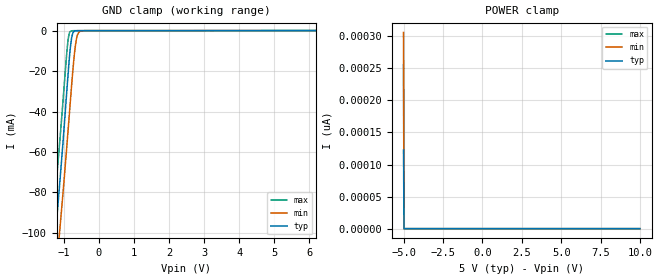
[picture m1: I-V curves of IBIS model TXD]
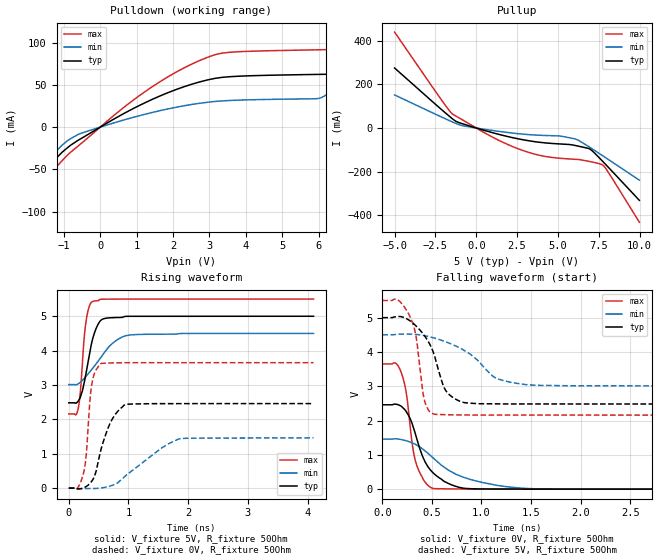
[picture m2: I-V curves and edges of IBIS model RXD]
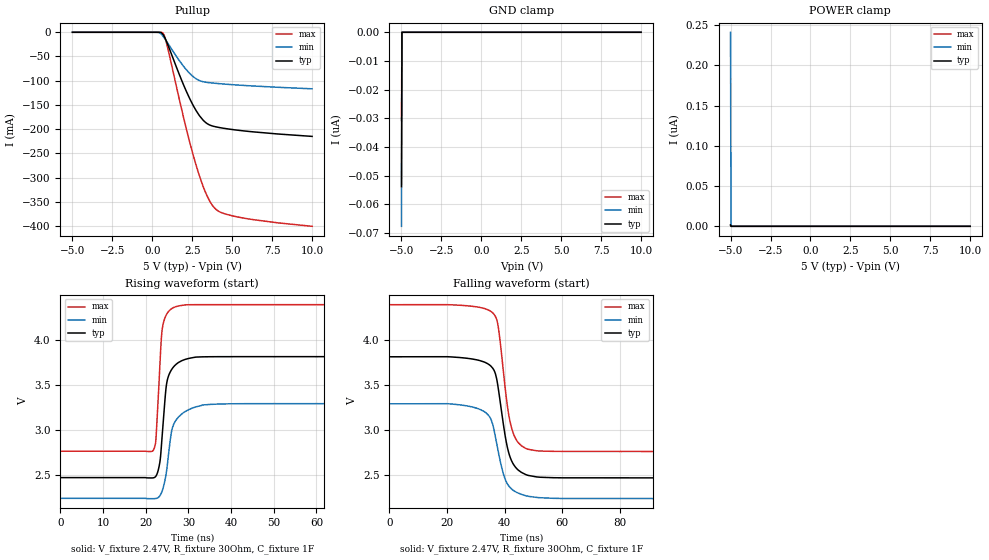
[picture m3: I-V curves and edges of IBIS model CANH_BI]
| Texas Instruments Incorporated
| CAN Transceiver Optimized for highly loaded networks
| Marketing part#   Voltage Range   Package-type   #pins/pkg drawing
| SN65HVD255D   4.5V - 5.5V   SOIC   8-pin D
[IBIS Ver]   4.0
[File name]   hvd255.ibs
[File Rev]   1.0
[Date]   05/01/2012
[Source]   Model built from TISPICED simulations at:
   Texas Instruments Incorporated.
   Analog-eLab, HPA
   12500 TI Blvd
   Dallas, TX -75243
   For Support e-mail: elab_ibis@list.ti.com
[Notes]   Revision History
   Rev 1.0: 05/01/2012
   - Initial model not matched to silicon
   - ccomp values are based on PVT settings:
   MIN: Low Voltage, High Temperature, Weak Process
   TYP: Nominal Voltage, Nominal Temperature, Nominal Process
   MAX: High Voltage, Low Temperature, Fast Process
   - User may change ccomp in the order of number values as
   per end simulator used
   - C_comp although listed in numberical order of value are obtained from varying PVT conditions.
   For PVT conditions for eachspecific value, refer to the buffer description under repective [Model].
   IBIS model user is responsible for using appropriate C_comp to simulate for Signal Integrity.
   - FAULT model not used on device HVD254
[Disclaimer] This model is designed as an aid for customers of Texas Instruments.
 TI and its licensors and suppliers make no warranties, either expressed
 or implied, with respect to this  model, including the warranties of
 merchantability or fitness for a particular purpose.
 The model is provided solely on an "as is" basis. The entire risk as to
 its quality and performance is with the customer.
[Copyright] (C)Copyright 2012 Texas Instruments Incorporated.
   All rights reserved.
|   Component HVD255D
[Component]   HVD255D
[Manufacturer]  Texas Instruments Incorporated
[Package]   |8-pin SOIC D package
|   typ   min   max
R_pkg   0.077174   0.00230   0.11690
L_pkg   2.321345nH   1.36253nH   2.80112nH
C_pkg   0.398513pF   0.31326pF   0.46592pF
[Pin] signal_name   model_name   R_pin   L_pin   C_pin
   1   TXD   TXD   0.11215   2.70023n   0.38408p
   2   GND   GND   0.03900   2.09764n   0.46592p
   3   VCC   POWER   0.02513   1.85198n   0.46577p
   4   RXD   RXD   0.11876   2.80112n   0.38992p
   5   NC   NC   0.00230   1.36253n   0.31326p
   6   CANL   CANL_BI   0.11690   2.72346n   0.40067p
   7   CANH   CANH_BI   0.09586   2.40528n   0.38694p
   8   S   S   0.10729   2.62852n   0.38154p
[Diff_pin]   inv_pin   vdiff   tdelay_typ   tdelay_min   tdelay_max
| The CANH and CANL are Diff_pins
7   6   0.9V   0 0 0
[Pin Mapping]pulldown_ref pullup_ref gnd_clamp_ref power_clamp_ref |ext_ref
1   NC   NC   GNDBUS1   PWRBUS1
2   GNDBUS1   NC
3   NC   PWRBUS1
4   GNDBUS1   PWRBUS1   GNDBUS1   PWRBUS1
5   NC   NC   NC   NC
6   GNDBUS1   NC   GNDBUS1   PWRBUS1  |CANL has no pullup
7   NC   PWRBUS1   GNDBUS1   PWRBUS1  |CANH has no pulldown
8   NC   NC   GNDBUS1   PWRBUS1
| Models and submodels in the file (6): TXD (Input), RXD (Output), CANH_BI (I/O_open_source), CANL_BI (I/O_open_drain), S (Input), FAULT (Open_drain)
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[Model]   TXD
Model_type   Input
Vinl = .8
Vinh = 2
|   typ   min   max
|   (nom PVT)   (fast PVT)   (slow PVT)
C_comp   3.6778e-13   3.5291e-13   3.9050e-13
[Voltage Range]   5   4.5   5.5
[Temperature Range]   27   125   -40
[Power Clamp Reference]   5   4.5   5.5
[GND Clamp Reference]   -0   -0   -0
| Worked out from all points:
|   GND clamp passes 1 mA (typ) near -0.73 V on its own axis
[GND Clamp]
|   Voltage   I(typ)   I(min)   I(max)
-5V       -570.9mA   -586.3mA   -524.8mA
-1.52V    -152.4mA   -171.3mA   -129.5mA
-1.25V    -104mA     -125.3mA   -83mA
-1.175V   -89.21mA   -111.5mA   -68.55mA
-1.1V     -73.64mA   -97.17mA   -53.22mA
-890mV    -25.89mA   -53.52mA   -7.625mA
-845mV    -15.82mA   -43.57mA   -1.999mA
-770mV    -3.617mA   -27.03mA   -122.8uA
-680mV    -194.6uA   -9.851mA   -56.54uA
-620mV    -44.75uA   -3.136mA   -55.35uA
-410mV    -27.79uA   -23.19uA   -55.14uA
9.985V    0A         0A         0A
[POWER Clamp]
|   Voltage   I(typ)   I(min)   I(max)
-5V       122.8pA    306.1pA    255.9pA
-4.97V    0A         0A         0A
-4.955V   0A         0A         0A
9.985V    0A         0A         0A
[Model]   RXD
Model_type   Output
Polarity   Non-Inverting
Vmeas = 2.5
Vref = 2.5
Cref = 15pF
Rref = 50
|   typ   min   max
|   (fast PVT)   (slow PVT)   (nom PVT)
C_comp   5.9114e-13   5.3173e-13   6.1323e-13
|C_comp (Low state)   4.8045e-13   4.1656e-13   4.9396e-13
[Voltage Range]   5   4.5   5.5
[Temperature Range]   27   125   -40
[Pullup Reference]   5   4.5   5.5
[Pulldown Reference]   -0   -0   -0
[Power Clamp Reference]   5   4.5   5.5
[GND Clamp Reference]   -0   -0   -0
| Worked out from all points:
|   slope of the pulldown table from 0 to 0.75 V, typ, clamps not added: 40.7 ohm
|   slope of the pullup table from 0 to 0.75 V, typ, clamps not added: 45.7 ohm
|   falling waveform, V_fixture 0V, R_fixture 50Ohm: 20-80 % time 213ps typ, 470ps min, 109ps max; typ from 2.46 V to 0 V
|   rising waveform, V_fixture 5V, R_fixture 50Ohm: 20-80 % time 179ps typ, 410ps min, 92.9ps max; typ from 2.48 V to 5 V
|   rising waveform, V_fixture 0V, R_fixture 50Ohm: 20-80 % time 258ps typ, 648ps min, 99.1ps max; typ from 0 V to 2.46 V
|   falling waveform, V_fixture 5V, R_fixture 50Ohm: 20-80 % time 200ps typ, 391ps min, 102ps max; typ from 5 V to 2.48 V
[Pulldown]
|   Voltage   I(typ)   I(min)   I(max)
-5V       -332.5mA   -214.5mA   -493.8mA
-2.42V    -126.3mA   -86.2mA    -180mA
-1.91V    -86.33mA   -61.25mA   -119mA
-1.34V    -44.01mA   -34.12mA   -55.59mA
-905mV    -24.62mA   -16.3mA    -33.42mA
1.27V     29.7mA     15.69mA    43.2mA
2.95V     55.96mA    29.47mA    82.77mA
6.085V    62.56mA    35.09mA    91.73mA
6.805V    68.02mA    57.39mA    93.42mA
7.6V      116.5mA    84.88mA    127.3mA
8.02V     144mA      99.59mA    171.2mA
9.985V    274.3mA    169mA      383.7mA
[Pullup]
|   Voltage   I(typ)   I(min)   I(max)
-5V       275mA      151.6mA    439.7mA
-2.105V   83.19mA    49.72mA    126.1mA
-1.43V    40.51mA    26.77mA    62.81mA
-830mV    19.17mA    10.51mA    36.67mA
1.09V     -23.4mA    -12.38mA   -45.47mA
2.95V     -55.06mA   -28.62mA   -105.5mA
4.3V      -68.72mA   -34.42mA   -131.4mA
6.04V     -79.81mA   -50.03mA   -143.4mA
6.97V     -96.87mA   -89.43mA   -154mA
7.69V     -149mA     -124.7mA   -167.5mA
7.99V     -172.5mA   -139.6mA   -192.5mA
9.985V    -331.6mA   -238.9mA   -431.7mA
[Ramp]
R_load = 50
|   typ   min   max
dV/dt_r   1.51123/1.78766e-10   0.893325/4.10159e-10   2.00518/9.28523e-11
dV/dt_f   1.47539/2.13452e-10   0.875752/4.70164e-10   2.18933/1.08841e-10
[Falling Waveform]
V_fixture = 0V
V_fixture_min = 0V
V_fixture_max = 0V
R_fixture = 50Ohm
C_fixture = 0F
|   Time   V(typ)   V(min)   V(max)
0s        2.459V     1.46V      3.649V
182.6ps   2.431V     1.451V     3.465V
240.9ps   2.26V      1.41V      2.821V
302.7ps   1.892V     1.347V     1.297V
339.8ps   1.546V     1.298V     761.2mV
430.9ps   797.4mV    1.115V     206.5mV
508.6ps   486mV      921.1mV    24.56mV
776.4ps   51.94mV    396.4mV    6.195mV
1.358ns   2.926mV    41.42mV    1.836mV
4.1ns     753.2nV    7.306uV    39.32uV
[Rising Waveform]
V_fixture = 5V
V_fixture_min = 4.5V
V_fixture_max = 5.5V
R_fixture = 50Ohm
C_fixture = 0F
|   Time   V(typ)   V(min)   V(max)
0s        2.481V     3.011V     2.158V
118.6ps   2.471V     3.007V     2.132V
159.6ps   2.536V     3.035V     2.322V
205.6ps   2.71V      3.097V     3.037V
278ps     3.237V     3.228V     4.707V
327.4ps   3.706V     3.331V     5.193V
393.1ps   4.291V     3.47V      5.424V
549.1ps   4.899V     3.829V     5.496V
1.031ns   4.999V     4.457V     5.5V
4.1ns     5V         4.5V       5.5V
[Rising Waveform]
V_fixture = 0V
V_fixture_min = 0V
V_fixture_max = 0V
R_fixture = 50Ohm
C_fixture = 0F
|   Time   V(typ)   V(min)   V(max)
0s        45.42nV    2.376nV    39.3uV
141.6ps   -22.31mV   -10.7mV    -8.758mV
240.9ps   890.1uV    -13.85mV   394.4mV
290.4ps   43.88mV    -13.49mV   923.9mV
381.8ps   192.3mV    -12.84mV   2.975V
530.8ps   1.063V     677.6uV    3.619V
707.8ps   1.942V     68mV       3.642V
966.7ps   2.437V     381.7mV    3.648V
1.848ns   2.458V     1.431V     3.648V
4.1ns     2.459V     1.46V      3.649V
[Falling Waveform]
|Gnd
V_fixture = 5V
V_fixture_min = 4.5V
V_fixture_max = 5.5V
R_fixture = 50Ohm
C_fixture = 0F
|   Time   V(typ)   V(min)   V(max)
0s        5V         4.5V       5.5V
278ps     4.909V     4.521V     5.038V
339.8ps   4.758V     4.51V      4.462V
427.4ps   4.465V     4.473V     2.56V
519.9ps   3.941V     4.41V      2.189V
629.7ps   2.924V     4.306V     2.171V
825.4ps   2.523V     4.046V     2.163V
1.143ns   2.487V     3.244V     2.16V
1.453ns   2.484V     3.046V     2.159V
4.1ns     2.481V     3.011V     2.158V
[Model]   CANH_BI
Model_type   I/O_open_source
Polarity   Non-Inverting
Vinl = 0.5V
Vinh = 0.9V
Vmeas = 2.47V
Vref = 2.47V
Rref = 30
|   typ   min   max
|   (nom PVT)   (slow PVT)   (fast PVT)
C_comp   9.760pF   8.703pF   11.05pF
|C_comp (ON state)   9.760pF   8.703pF   11.05pF
|   (nom PVT)   (fast PVT)   (slow PVT)
|C_comp (OFF state)   6.980pF   6.075pF   7.757pF
[Voltage Range]   5   4.5   5.5
[Temperature Range]   27   125   -40
[Pullup Reference]   5   4.5   5.5
[Pulldown Reference]   -0   -0   -0
[Power Clamp Reference]   5   4.5   5.5
[GND Clamp Reference]   -0   -0   -0
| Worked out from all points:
|   slope of the pullup table from 0 to 0.75 V, typ, clamps not added: 79.4 ohm
|   falling waveform, V_fixture 2.47V, R_fixture 30Ohm, C_fixture 1F: 20-80 % time 4.14ns typ, 4.59ns min, 3.79ns max; typ from 3.81 V to 2.47 V
|   rising waveform, V_fixture 2.47V, R_fixture 30Ohm, C_fixture 1F: 20-80 % time 1.49ns typ, 2.21ns min, 1.12ns max; typ from 2.47 V to 3.81 V
[GND Clamp]
|   Voltage   I(typ)   I(min)   I(max)
-5V       -53.77nA   -67.62nA   -30.78nA
-4.97V    0A         0A         0A
-4.955V   0A         0A         0A
9.985V    0A         0A         0A
[Pullup]
|   Voltage   I(typ)   I(min)   I(max)
-5V       2.731pA    10.01pA    13.35pA
295mV     -935nA     -49.51uA   -39.84nA
640mV     -3.443mA   -7.065mA   -1.059mA
745mV     -9.123mA   -11.78mA   -7.02mA
850mV     -16.55mA   -16.85mA   -18.2mA
2.05V     -116.5mA   -74.46mA   -189.9mA
2.71V     -160.5mA   -95.5mA    -272.2mA
3.31V     -185.9mA   -103mA     -329.8mA
3.79V     -193.9mA   -104.9mA   -359.3mA
4.21V     -196.9mA   -106.2mA   -371mA
5.26V     -202mA     -108.8mA   -381mA
9.985V    -215mA     -116.8mA   -400.8mA
[POWER Clamp]
|   Voltage   I(typ)   I(min)   I(max)
-5V       1.667nA    240.9nA    1.137nA
-4.97V    0A         0A         0A
-4.955V   0A         0A         0A
9.985V    0A         0A         0A
[Ramp]
R_load = 30
|   typ   min   max
dV/dt_r   0.80562/1.48598e-09   0.630884/2.20577e-09   0.976191/1.12349e-09
dV/dt_f   0.805534/4.14379e-09   0.630773/4.56735e-09   0.976122/3.7928e-09
[Falling Waveform]
V_fixture = 2.47V
V_fixture_min = 2.24V
V_fixture_max = 2.763V
R_fixture = 30Ohm
C_fixture = 1F
|   Time   V(typ)   V(min)   V(max)
0s        3.813V     3.291V     4.39V
28.4ns    3.79V      3.259V     4.374V
33.4ns    3.748V     3.194V     4.343V
36ns      3.68V      3.046V     4.295V
37.9ns    3.44V      2.745V     4.119V
40.3ns    2.917V     2.448V     3.437V
42.2ns    2.676V     2.354V     3.051V
44.4ns    2.567V     2.307V     2.876V
47.8ns    2.502V     2.269V     2.791V
139.9ns   2.47V      2.24V      2.763V
[Rising Waveform]
V_fixture = 2.47V
V_fixture_min = 2.24V
V_fixture_max = 2.763V
R_fixture = 30Ohm
C_fixture = 1F
|   Time   V(typ)   V(min)   V(max)
0s        2.47V      2.24V      2.763V
21.7ns    2.467V     2.236V     2.77V
22.4ns    2.488V     2.239V     2.908V
23.3ns    2.64V      2.268V     3.71V
23.9ns    2.97V      2.33V      4.131V
25ns      3.541V     2.59V      4.292V
26.1ns    3.673V     2.995V     4.347V
27.5ns    3.742V     3.133V     4.374V
37.6ns    3.813V     3.287V     4.39V
139.9ns   3.813V     3.291V     4.39V
